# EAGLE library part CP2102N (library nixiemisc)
USB to UART converter with battery charging detection
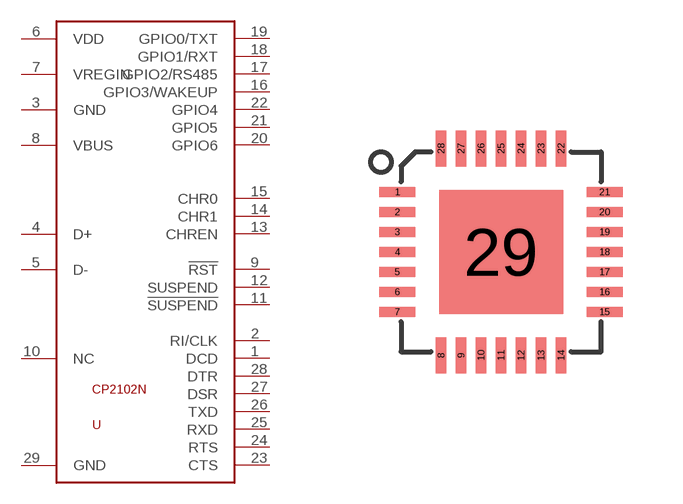
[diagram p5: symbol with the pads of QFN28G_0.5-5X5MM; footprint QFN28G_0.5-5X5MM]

Designator prefix U

## CP2102N  [QFN28G_0.5-5X5MM]
1  DCD  in
2  RI/CLK
3  GND  pwr
4  D+  in
5  D-  in
6  VDD  pwr
7  VREGIN  pwr
8  VBUS  pwr
9  !RST!
10  NC  nc
11  !SUSPEND!  out
12  SUSPEND  out
13  CHREN  out
14  CHR1  out
15  CHR0  out
16  GPIO3/WAKEUP
17  GPIO2/RS485
18  GPIO1/RXT
19  GPIO0/TXT
20  GPIO6
21  GPIO5
22  GPIO4
23  CTS  in
24  RTS  out
25  RXD  in
26  TXD  out
27  DSR  in
28  DTR  out
29  GND  pwr

## Footprint QFN28G_0.5-5X5MM (pad centres in mm)
smd 0.9 x 0.254: 1 -2.59,1.5; 2 -2.59,1; 3 -2.59,0.5; 4 -2.59,0; 5 -2.59,-0.5; 6 -2.59,-1; 7 -2.59,-1.5; 15 2.59,-1.5; 16 2.59,-1; 17 2.59,-0.5; 18 2.59,0; 19 2.59,0.5; 20 2.59,1; 21 2.59,1.5
smd 0.254 x 0.9: 8 -1.5,-2.59; 9 -1,-2.59; 10 -0.5,-2.59; 11 0,-2.59; 12 0.5,-2.59; 13 1,-2.59; 14 1.5,-2.59; 22 1.5,2.59; 23 1,2.59; 24 0.5,2.59; 25 0,2.59; 26 -0.5,2.59; 27 -1,2.59; 28 -1.5,2.59
smd 3.1 x 3.1: 29 0,0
